ORGANIZATION_BLOCK "Hardware Interrupt 6"
TITLE =
VERSION : 0.1


VAR_TEMP
  OB46_EV_CLASS : BYTE ;	//Bits 0-3 = 1 (Coming event), Bits 4-7 = 1 (Event class 1)
  OB46_STRT_INF : BYTE ;	//16#41/42/43/44 (Interrupt 1/2/3/4)
  OB46_PRIORITY : BYTE ;	//22 (Priority of 1 is lowest)
  OB46_OB_NUMBR : BYTE ;	//46 (Organization block 46, OB46)
  OB46_RESERVED_1 : BYTE ;	//Reserved for system
  OB46_RESERVED_2 : BYTE ;	//Reserved for system
  OB46_MDL_ADDR : WORD ;	//Base address of module initiating interrupt
  OB46_POINT_ADDR : DWORD ;	//Address of interrupt point on module
  OB46_DATE_TIME : DATE_AND_TIME ;	//Date and time OB46 started
END_VAR
BEGIN
END_ORGANIZATION_BLOCK

